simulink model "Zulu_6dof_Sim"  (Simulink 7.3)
settings: Solver=ode45  StartTime=0.0  StopTime=315  RelTol=1e-4
InitFcn:
  | init
StopFcn:
  | pl
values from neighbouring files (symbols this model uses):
  accel = [-225, 0, 0]    [init.m]
  ch = 7.761    [init.m]
  d2r = pi/180    (= 0.0174532925199)    [init.m]    (also in pl.m; run.m; LQR_Des.m)
  Euler_0 = [0, 49.766, 0]*d2r    [init.m]
  h0 = 43031    [init.m]
  Ixxpr = ee*Zulu_Mass(:,2)    [init.m]
  Ixypr = ee*Zulu_Mass(:,5)    [init.m]
  Ixzpr = ee*Zulu_Mass(:,6)    [init.m]
  Iyypr = ee*Zulu_Mass(:,3)    [init.m]
  Iyzpr = ee*Zulu_Mass(:,7)    [init.m]
  Izzpr = ee*Zulu_Mass(:,4)    [init.m]
  mrc = [x_ref, y_ref, z_ref]    [init.m]
  msspr = ee*Zulu_Mass(:,1)    [init.m]
  r2d = 180/pi    (= 57.2957795131)    [init.m]    (also in pl.m; run.m; LQR_Des.m)
  rcs1 = [-120.0, -4.0, -0.0]    [init.m]
  rcs2 = [-120.0, +4.0, -0.0]    [init.m]
  sp = 7.761    [init.m]
  Sref = 47.308    [init.m]
  Tst2 = 170.0    (= 170)    [init.m]
  Tstg = 91.2    [init.m]
  tvc1 = [-244.6, -8.7, 0.0]    [init.m]
  tvc2 = [-244.6, +8.7, 0.0]    [init.m]
  tvc3 = [-244.6,  0.0, 0.0]    [init.m]
  tvc4 = [-200.0, 0.0, 0.06]    [init.m]
  Xcgpr = ee*Zulu_Mass(:,8)    [init.m]
  Ycgpr = ee*Zulu_Mass(:,9)    [init.m]
  Zcgpr = ee*Zulu_Mass(:,10)    [init.m]
undefined symbols (not defined in the file or in its folder): Cl, Cl2, Cm, Cm2, Cn, Cn2, Continuous, CX, CX2, CY, CY2, CZ, CZ2, Dryden, Earth, F, ft, km, Light, MIL, q, r, sigbuilder_block, STD, WGS84
libraries: aerolibutil x7, aerolibasang x3, aerolibwind2 x3, aerolibactuator x2, aerolibconvert2 x1, aerolibatmos2 x1, aerolibgravity2 x1, aerolibadyn x1, aerolib6dof2 x1
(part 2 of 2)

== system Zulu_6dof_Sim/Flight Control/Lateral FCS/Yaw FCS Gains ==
  Demux : Demux  Tag=STV Demux  Outputs=6
  FromWs : FromWorkspace  Tag=STV FromWs  VariableName=tuvar  SampleTime=0  SigBuilderData=DataTag6  VnvData=DataTag7
  Kml3 : Outport  Tag=STV Outport
  Kr_phi : Outport  Tag=STV Outport  Port=2
  Kr_p : Outport  Tag=STV Outport  Port=3
  Kr_psi : Outport  Tag=STV Outport  Port=4
  Kr_r : Outport  Tag=STV Outport  Port=5
  Kr_beta : Outport  Tag=STV Outport  Port=6
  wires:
  FromWs/1 -> Demux/1
  Demux/1 -> Kml3/1
  Demux/2 -> Kr_phi/1
  Demux/3 -> Kr_p/1
  Demux/4 -> Kr_psi/1
  Demux/5 -> Kr_r/1
  Demux/6 -> Kr_beta/1

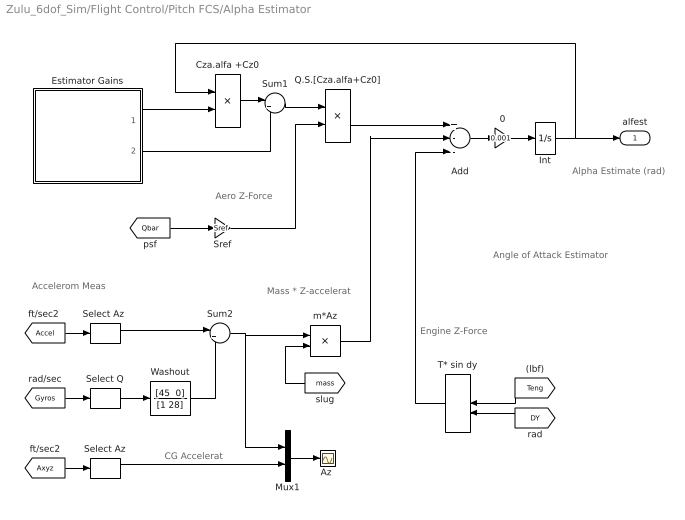
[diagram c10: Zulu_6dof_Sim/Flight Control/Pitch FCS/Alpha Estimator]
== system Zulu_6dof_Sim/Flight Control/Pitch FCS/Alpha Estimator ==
  note: Angle of Attack Estimator
  note: Engine Z-Force
  note: Aero Z-Force
  note: Mass * Z-accelerat
  note: Alpha Estimate (rad)
  note: Accelerom Meas
  note: CG Accelerat
  0 : Gain  Gain=0.001  ParameterDataType=sfix(16)  ParameterScaling=2^0  OutDataType=sfix(16)  OutScaling=2^0
  Add : Sum  Inputs=+--  OutDataType=fixdt(1, 16)  OutScaling=2^-10
  "Az " : Scope
  Cza.alfa +Cz0 : Product  OutDataType=fixdt(1, 16)  OutScaling=2^0
  Estimator Gains : Subsystem  Tag=STV Subsys  LoadFcn=sigbuilder_block('load');  StartFcn=sigbuilder_block('start');  StopFcn=sigbuilder_block('stop');  ClipboardFcn=sigbuilder_block('clipboard');
  Int : Integrator
  Mux1 : Mux  Inputs=2
  Q.S.[Cza.alfa+Cz0] : Product  OutDataType=fixdt(1, 16)  OutScaling=2^0
  Select Az : Selector  InputPortWidth=3  IndexOptions=Index vector (dialog)  Indices=[3]  OutputSizes=1
  "Select Az " : Selector  InputPortWidth=3  IndexOptions=Index vector (dialog)  Indices=[3]  OutputSizes=1
  Select Q : Selector  InputPortWidth=3  IndexOptions=Index vector (dialog)  Indices=[2]  OutputSizes=1
  Sref : Gain  Gain=Sref  ParameterDataType=sfix(16)  ParameterScaling=2^0  OutDataType=sfix(16)  OutScaling=2^0
  Sum1 : Sum  Inputs=|++  OutDataType=fixdt(1, 16)  OutScaling=2^0
  Sum2 : Sum  Inputs=|++  OutDataType=fixdt(1, 16)  OutScaling=2^0
  T* sin dy : DotProduct  OutDataType=fixdt(1, 16)  OutScaling=2^-10
  Washout : TransferFcn  Numerator="[45  0]"  Denominator=[1 28]
  m*Az : Product  OutDataType=fixdt(1, 16)  OutScaling=2^0
  alfest : Outport
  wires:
  [DY] -> T* sin dy/2
  [Teng] -> T* sin dy/1
  [mass] -> m*Az/2
  [Qbar] -> Sref/1
  Int/1 -> Cza.alfa +Cz0/1, alfest/1
  Estimator Gains/1(Cz_alpha) -> Cza.alfa +Cz0/2
  Cza.alfa +Cz0/1 -> Sum1/1
  Sum1/1 -> Q.S.[Cza.alfa+Cz0]/1
  Sref/1 -> Q.S.[Cza.alfa+Cz0]/2
  Q.S.[Cza.alfa+Cz0]/1 -> Add/1
  Add/1 -> 0/1
  Estimator Gains/2(CZ0) -> Sum1/2
  m*Az/1 -> Add/2
  T* sin dy/1 -> Add/3
  0/1 -> Int/1
  Mux1/1 -> "Az "/1
  [Gyros] -> Select Q/1
  Select Q/1 -> Washout/1
  Sum2/1 -> m*Az/1, Mux1/1
  [Axyz] -> Select Az/1
  [Accel] -> "Select Az "/1
  "Select Az "/1 -> Sum2/1
  Select Az/1 -> Mux1/2
  Washout/1 -> Sum2/2

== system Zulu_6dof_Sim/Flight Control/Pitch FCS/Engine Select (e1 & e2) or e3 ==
  note: Stage-1
  note: Stage-2
  "DY " : Inport
  Clock : Clock
  Mux : Mux  Inputs=3
  Switch : Switch  Threshold=Tstg  OutDataType=fixdt(1, 16)  OutScaling=2^0
  Switch1 : Switch  Threshold=Tstg  OutDataType=fixdt(1, 16)  OutScaling=2^0
  grd : Ground
  DY : Outport
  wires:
  Clock/1 -> Switch/2, Switch1/2
  "DY "/1 -> Switch1/1, Switch/3
  Switch/1 -> Mux/1, Mux/2
  Switch1/1 -> Mux/3
  grd/1 -> Switch1/3, Switch/1
  Mux/1 -> DY/1

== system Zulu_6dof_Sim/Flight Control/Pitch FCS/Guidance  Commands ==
  Demux : Demux  Tag=STV Demux  Outputs=2
  FromWs : FromWorkspace  Tag=STV FromWs  VariableName=tuvar  SampleTime=0  SigBuilderData=DataTag10  VnvData=DataTag11
  Theta_cmd : Outport  Tag=STV Outport
  Gamma_cmd : Outport  Tag=STV Outport  Port=2
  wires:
  Demux/2 -> Gamma_cmd/1
  Demux/1 -> Theta_cmd/1
  FromWs/1 -> Demux/1

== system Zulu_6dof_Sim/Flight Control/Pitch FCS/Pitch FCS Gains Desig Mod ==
  Demux : Demux  Tag=STV Demux  Outputs=5
  FromWs : FromWorkspace  Tag=STV FromWs  VariableName=tuvar  SampleTime=0  SigBuilderData=DataTag12  VnvData=DataTag13
  Kml2 : Outport  Tag=STV Outport
  Kq_theta : Outport  Tag=STV Outport  Port=2
  Kq_gam_int : Outport  Tag=STV Outport  Port=3
  Kq_q : Outport  Tag=STV Outport  Port=4
  Kq_alpha : Outport  Tag=STV Outport  Port=5
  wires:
  FromWs/1 -> Demux/1
  Demux/1 -> Kml2/1
  Demux/2 -> Kq_theta/1
  Demux/3 -> Kq_gam_int/1
  Demux/4 -> Kq_q/1
  Demux/5 -> Kq_alpha/1

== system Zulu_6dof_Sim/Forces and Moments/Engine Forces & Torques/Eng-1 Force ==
  note: Engine Force
  Thrust : Inport
  dy : Inport  Port=2
  dz : Inport  Port=3
  -1 : Gain  Gain=-1  ParameterDataType=sfix(16)  ParameterScaling=2^0  OutDataType=sfix(16)  OutScaling=2^0
  Fx1 : Product  Inputs=3  OutDataType=fixdt(1, 16)  OutScaling=2^0
  Fy1 : Product  Inputs=3  OutDataType=fixdt(1, 16)  OutScaling=2^0
  Fz1 : Product  OutDataType=fixdt(1, 16)  OutScaling=2^0
  Mux : Mux  Inputs=3
  cos(dy) : Trigonometry  Operator=cos
  cos(dz) : Trigonometry  Operator=cos
  sin(dy) : Trigonometry
  sin(dz) : Trigonometry
  F1 : Outport  OutDataType=sfix(16)  OutScaling=2^0  InitialOutput=0
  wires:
  dz/1 -> sin(dz)/1, cos(dz)/1
  dy/1 -> sin(dy)/1, cos(dy)/1
  sin(dy)/1 -> Fz1/2
  sin(dz)/1 -> Fy1/3
  cos(dz)/1 -> Fx1/3
  Mux/1 -> F1/1
  Fx1/1 -> Mux/1
  Fz1/1 -> Mux/3
  Fy1/1 -> Mux/2
  -1/1 -> Fz1/1
  cos(dy)/1 -> Fx1/2, Fy1/2
  Thrust/1 -> Fx1/1, Fy1/1, -1/1

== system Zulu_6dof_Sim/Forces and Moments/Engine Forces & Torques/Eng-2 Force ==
  note: Engine Force
  Thrust : Inport
  dy : Inport  Port=2
  dz : Inport  Port=3
  -1 : Gain  Gain=-1  ParameterDataType=sfix(16)  ParameterScaling=2^0  OutDataType=sfix(16)  OutScaling=2^0
  Fx1 : Product  Inputs=3  OutDataType=fixdt(1, 16)  OutScaling=2^0
  Fy1 : Product  Inputs=3  OutDataType=fixdt(1, 16)  OutScaling=2^0
  Fz1 : Product  OutDataType=fixdt(1, 16)  OutScaling=2^0
  Mux : Mux  Inputs=3
  cos(dy) : Trigonometry  Operator=cos
  cos(dz) : Trigonometry  Operator=cos
  sin(dy) : Trigonometry
  sin(dz) : Trigonometry
  F1 : Outport  OutDataType=sfix(16)  OutScaling=2^0  InitialOutput=0
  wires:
  dz/1 -> sin(dz)/1, cos(dz)/1
  dy/1 -> sin(dy)/1, cos(dy)/1
  sin(dy)/1 -> Fz1/2
  sin(dz)/1 -> Fy1/3
  cos(dz)/1 -> Fx1/3
  Mux/1 -> F1/1
  Fx1/1 -> Mux/1
  Fz1/1 -> Mux/3
  Fy1/1 -> Mux/2
  -1/1 -> Fz1/1
  cos(dy)/1 -> Fx1/2, Fy1/2
  Thrust/1 -> Fx1/1, Fy1/1, -1/1

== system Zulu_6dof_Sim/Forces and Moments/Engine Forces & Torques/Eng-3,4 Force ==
  note: Engine Force
  Thrust : Inport
  dy : Inport  Port=2
  dz : Inport  Port=3
  -1 : Gain  Gain=-1  ParameterDataType=sfix(16)  ParameterScaling=2^0  OutDataType=sfix(16)  OutScaling=2^0
  Fx1 : Product  Inputs=3  OutDataType=fixdt(1, 16)  OutScaling=2^0
  Fy1 : Product  Inputs=3  OutDataType=fixdt(1, 16)  OutScaling=2^0
  Fz1 : Product  OutDataType=fixdt(1, 16)  OutScaling=2^0
  Mux : Mux  Inputs=3
  cos(dy) : Trigonometry  Operator=cos
  cos(dz) : Trigonometry  Operator=cos
  sin(dy) : Trigonometry
  sin(dz) : Trigonometry
  F1 : Outport  OutDataType=sfix(16)  OutScaling=2^0  InitialOutput=0
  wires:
  dz/1 -> sin(dz)/1, cos(dz)/1
  dy/1 -> sin(dy)/1, cos(dy)/1
  sin(dy)/1 -> Fz1/2
  sin(dz)/1 -> Fy1/3
  cos(dz)/1 -> Fx1/3
  Mux/1 -> F1/1
  Fx1/1 -> Mux/1
  Fz1/1 -> Mux/3
  Fy1/1 -> Mux/2
  -1/1 -> Fz1/1
  cos(dy)/1 -> Fx1/2, Fy1/2
  Thrust/1 -> Fx1/1, Fy1/1, -1/1

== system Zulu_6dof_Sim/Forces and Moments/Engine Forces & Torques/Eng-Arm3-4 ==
  Clock : Clock
  Switch : Switch  Threshold=169.9  OutDataType=fixdt(1, 16)  OutScaling=2^0
  lg3 : Outport
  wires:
  Clock/1 -> Switch/2
  [lg4] -> Switch/1
  [lg3] -> Switch/3
  Switch/1 -> lg3/1

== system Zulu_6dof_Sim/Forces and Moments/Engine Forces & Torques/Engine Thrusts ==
  Demux : Demux  Tag=STV Demux  Outputs=3
  FromWs : FromWorkspace  Tag=STV FromWs  VariableName=tuvar  SampleTime=0  SigBuilderData=DataTag14  VnvData=DataTag15
  Thrust-1 : Outport  Tag=STV Outport
  Thrust-2 : Outport  Tag=STV Outport  Port=2
  Thrust-3 : Outport  Tag=STV Outport  Port=3
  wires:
  FromWs/1 -> Demux/1
  Demux/1 -> Thrust-1/1
  Demux/2 -> Thrust-2/1
  Demux/3 -> Thrust-3/1

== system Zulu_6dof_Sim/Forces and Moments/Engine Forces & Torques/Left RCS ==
  note: RCS Force
  Thrust : Inport
  -1 : Gain  Gain=-1  ParameterDataType=sfix(16)  ParameterScaling=2^0  OutDataType=sfix(16)  OutScaling=2^0
  Fx1 : Product  Inputs=3  OutDataType=fixdt(1, 16)  OutScaling=2^0
  Fy1 : Product  Inputs=3  OutDataType=fixdt(1, 16)  OutScaling=2^0
  Fz1 : Product  OutDataType=fixdt(1, 16)  OutScaling=2^0
  Mux : Mux  Inputs=3
  cos(dy) : Trigonometry  Operator=cos
  cos(dz) : Trigonometry  Operator=cos
  dy=-90 : Constant  Value=-90*d2r  OutDataType=fixdt(1, 16)  OutScaling=2^0
  dz=0 : Constant  Value=0  OutDataType=fixdt(1, 16)  OutScaling=2^0
  sin(dy) : Trigonometry
  sin(dz) : Trigonometry
  FL : Outport  OutDataType=sfix(16)  OutScaling=2^0  InitialOutput=0
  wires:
  Thrust/1 -> -1/1, Fy1/1, Fx1/1
  cos(dy)/1 -> Fy1/2, Fx1/2
  -1/1 -> Fz1/1
  Fy1/1 -> Mux/2
  Fz1/1 -> Mux/3
  Fx1/1 -> Mux/1
  Mux/1 -> FL/1
  cos(dz)/1 -> Fx1/3
  sin(dz)/1 -> Fy1/3
  sin(dy)/1 -> Fz1/2
  dy=-90/1 -> cos(dy)/1, sin(dy)/1
  dz=0/1 -> cos(dz)/1, sin(dz)/1

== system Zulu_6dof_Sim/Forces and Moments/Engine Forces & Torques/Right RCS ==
  note: RCS Force
  Thrust : Inport
  -1 : Gain  Gain=-1  ParameterDataType=sfix(16)  ParameterScaling=2^0  OutDataType=sfix(16)  OutScaling=2^0
  Fx1 : Product  Inputs=3  OutDataType=fixdt(1, 16)  OutScaling=2^0
  Fy1 : Product  Inputs=3  OutDataType=fixdt(1, 16)  OutScaling=2^0
  Fz1 : Product  OutDataType=fixdt(1, 16)  OutScaling=2^0
  Mux : Mux  Inputs=3
  cos(dy) : Trigonometry  Operator=cos
  cos(dz) : Trigonometry  Operator=cos
  dy=-90 : Constant  Value=-90*d2r  OutDataType=fixdt(1, 16)  OutScaling=2^0
  dz=0 : Constant  Value=0  OutDataType=fixdt(1, 16)  OutScaling=2^0
  sin(dy) : Trigonometry
  sin(dz) : Trigonometry
  FL : Outport  OutDataType=sfix(16)  OutScaling=2^0  InitialOutput=0
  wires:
  Thrust/1 -> -1/1, Fy1/1, Fx1/1
  cos(dy)/1 -> Fy1/2, Fx1/2
  -1/1 -> Fz1/1
  Fy1/1 -> Mux/2
  Fz1/1 -> Mux/3
  Fx1/1 -> Mux/1
  Mux/1 -> FL/1
  cos(dz)/1 -> Fx1/3
  sin(dz)/1 -> Fy1/3
  sin(dy)/1 -> Fz1/2
  dy=-90/1 -> cos(dy)/1, sin(dy)/1
  dz=0/1 -> cos(dz)/1, sin(dz)/1

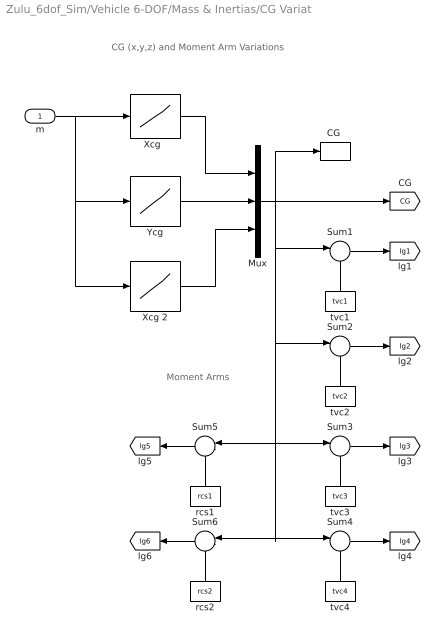
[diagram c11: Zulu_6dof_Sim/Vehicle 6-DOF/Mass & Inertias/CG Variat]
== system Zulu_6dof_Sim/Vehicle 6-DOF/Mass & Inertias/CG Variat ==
  note: CG (x,y,z) and Moment Arm Variations
  note: Moment Arms
  m : Inport
  "CG " : ToWorkspace  VariableName=CG  SampleTime=-1  SaveFormat=Array
  Mux : Mux  Inputs=3
  Sum{1..6} (6 alike) : Sum  Inputs=|-+  OutDataType=fixdt(1, 16)  OutScaling=2^0
  "Xcg  " : Lookup  InputValues=msspr  Table=Xcgpr  OutDataType=fixdt(1, 16)  OutScaling=2^0
  Xcg 2 : Lookup  InputValues=msspr  Table=Zcgpr  OutDataType=fixdt(1, 16)  OutScaling=2^0
  Ycg : Lookup  InputValues=msspr  Table=Ycgpr  OutDataType=fixdt(1, 16)  OutScaling=2^0
  rcs1 : Constant  Value=rcs1  OutDataType=fixdt(1, 16)  OutScaling=2^0
  rcs2 : Constant  Value=rcs2  OutDataType=fixdt(1, 16)  OutScaling=2^0
  tvc1 : Constant  Value=tvc1  OutDataType=fixdt(1, 16)  OutScaling=2^0
  tvc2 : Constant  Value=tvc2  OutDataType=fixdt(1, 16)  OutScaling=2^0
  tvc3 : Constant  Value=tvc3  OutDataType=fixdt(1, 16)  OutScaling=2^0
  tvc4 : Constant  Value=tvc4  OutDataType=fixdt(1, 16)  OutScaling=2^0
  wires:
  m/1 -> "Xcg  "/1, Ycg/1, Xcg 2/1
  Ycg/1 -> Mux/2
  Xcg 2/1 -> Mux/3
  "Xcg  "/1 -> Mux/1
  Mux/1 -> [CG], Sum1/1, Sum2/1, Sum3/1, Sum5/1, Sum4/1, Sum6/1, "CG "/1
  Sum1/1 -> [lg1]
  tvc1/1 -> Sum1/2
  tvc2/1 -> Sum2/2
  Sum2/1 -> [lg2]
  tvc3/1 -> Sum3/2
  Sum3/1 -> [lg3]
  tvc4/1 -> Sum4/2
  Sum4/1 -> [lg4]
  rcs1/1 -> Sum5/2
  rcs2/1 -> Sum6/2
  Sum5/1 -> [lg5]
  Sum6/1 -> [lg6]

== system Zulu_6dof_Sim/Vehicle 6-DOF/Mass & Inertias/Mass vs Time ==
  Demux : Demux  Tag=STV Demux  Outputs=1
  FromWs : FromWorkspace  Tag=STV FromWs  VariableName=tuvar  SampleTime=0  SigBuilderData=DataTag16  VnvData=DataTag17
  Mass (slg) : Outport  Tag=STV Outport
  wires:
  FromWs/1 -> Demux/1
  Demux/1 -> Mass (slg)/1

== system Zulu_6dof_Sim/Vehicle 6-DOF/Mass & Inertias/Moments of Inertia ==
  note: Moments and Products of Inertia as a Function of Mass
  mass : Inport
  "Inertias " : ToWorkspace  VariableName=MOI  SampleTime=-1  SaveFormat=Array
  "Ixx " : Lookup  InputValues=msspr  Table=Ixxpr  OutDataType=fixdt(1, 16)  OutScaling=2^0
  "Ixy " : Lookup  InputValues=msspr  Table=Ixypr  OutDataType=fixdt(1, 16)  OutScaling=2^0
  "Ixz " : Lookup  InputValues=msspr  Table=Ixzpr  OutDataType=fixdt(1, 16)  OutScaling=2^0
  "Iyy " : Lookup  InputValues=msspr  Table=Iyypr  OutDataType=fixdt(1, 16)  OutScaling=2^0
  "Iyz " : Lookup  InputValues=msspr  Table=Iyzpr  OutDataType=fixdt(1, 16)  OutScaling=2^0
  "Izz " : Lookup  InputValues=msspr  Table=Izzpr  OutDataType=fixdt(1, 16)  OutScaling=2^0
  Mux : Mux  Inputs=3
  Ixx : Outport
  Iyy : Outport  Port=2
  Izz : Outport  Port=3
  Ixy : Outport  Port=4
  Ixz : Outport  Port=5
  Iyz : Outport  Port=6
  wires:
  mass/1 -> "Ixx "/1, "Iyy "/1, "Izz "/1, "Ixy "/1, "Ixz "/1, "Iyz "/1
  "Ixx "/1 -> Ixx/1, Mux/1
  "Iyy "/1 -> Iyy/1, Mux/2
  "Izz "/1 -> Izz/1, Mux/3
  "Ixy "/1 -> Ixy/1
  "Ixz "/1 -> Ixz/1
  "Iyz "/1 -> Iyz/1
  Mux/1 -> "Inertias "/1

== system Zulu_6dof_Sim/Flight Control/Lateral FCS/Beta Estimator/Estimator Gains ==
  Demux : Demux  Tag=STV Demux  Outputs=1
  FromWs : FromWorkspace  Tag=STV FromWs  VariableName=tuvar  SampleTime=0  SigBuilderData=DataTag0  VnvData=DataTag1
  Cy_beta : Outport  Tag=STV Outport
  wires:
  Demux/1 -> Cy_beta/1
  FromWs/1 -> Demux/1

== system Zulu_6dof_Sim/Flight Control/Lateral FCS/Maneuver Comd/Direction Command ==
  Demux : Demux  Tag=STV Demux  Outputs=1
  FromWs : FromWorkspace  Tag=STV FromWs  VariableName=tuvar  SampleTime=0  SigBuilderData=DataTag2  VnvData=DataTag3
  Direct Cmd : Outport  Tag=STV Outport
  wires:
  FromWs/1 -> Demux/1
  Demux/1 -> Direct Cmd/1

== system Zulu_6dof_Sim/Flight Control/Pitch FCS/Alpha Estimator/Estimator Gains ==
  Demux : Demux  Tag=STV Demux  Outputs=2
  FromWs : FromWorkspace  Tag=STV FromWs  VariableName=tuvar  SampleTime=0  SigBuilderData=DataTag8  VnvData=DataTag9
  Cz_alpha : Outport  Tag=STV Outport
  CZ0 : Outport  Tag=STV Outport  Port=2
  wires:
  Demux/2 -> CZ0/1
  Demux/1 -> Cz_alpha/1
  FromWs/1 -> Demux/1
